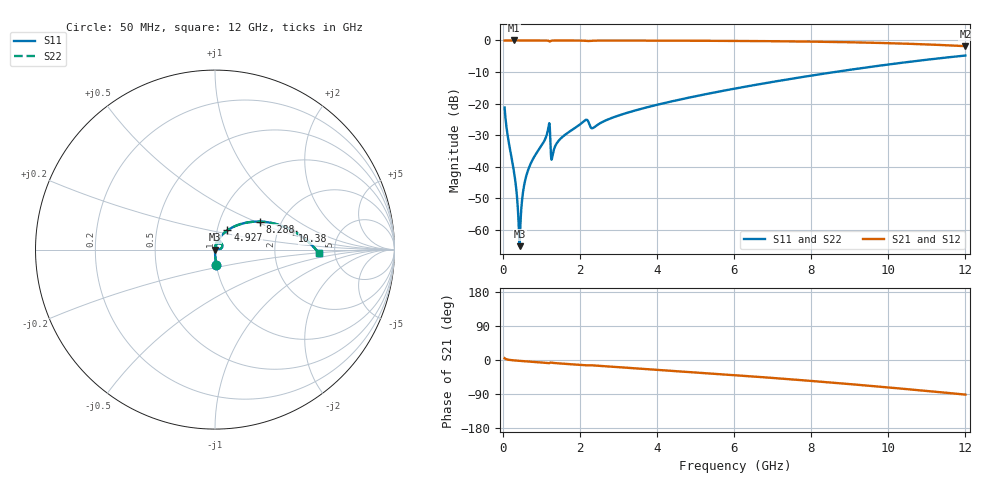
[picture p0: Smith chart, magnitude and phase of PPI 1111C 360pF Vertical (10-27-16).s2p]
# GHz S MA R 50
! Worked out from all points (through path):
!   1601 points, 50 MHz to 12 GHz, reference 50 ohm
!   highest |S21| = 0.00 dB at 289 MHz (marker M1); lowest = -1.8 dB at 12 GHz (marker M2)
!   group delay of S21, straight-line fit = 21 ps
!   lowest |S11| = -65.1 dB at 438.4 MHz (marker M3), VSWR 1.00, Z = 50.1 + j0.00672 ohm
!   |S11| at or under -10 dB: start of sweep to 8.61 GHz
!   |S22| runs from -65.1 to -4.8 dB; largest |S21 - S12| = 0
!   S11 on the Smith chart (normalised r, x): 50 MHz: 1.00, -0.17; 4.927 GHz: 1.12, +0.24; 8.288 GHz: 1.56, +0.53; 10.38 GHz: 2.41, +0.63; 12 GHz: 3.72, -0.19
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0.05  0.08683 -85.1  0.996 4.7  0.996 4.7  0.08683 -85.1
0.289  0.008632 -87.9  0.9995 -1.0  0.9995 -1.0  0.008632 -87.9
0.3412812  0.005086 -85.9  0.9995 -1.5  0.9995 -1.5  0.005086 -85.9
0.3935625  0.00218 -78.0  0.9995 -1.9  0.9995 -1.9  0.00218 -78.0
0.438375  0.0005533 7.0  0.9994 -2.3  0.9994 -2.3  0.0005533 7.0
0.4757188  0.001856 69.7  0.9994 -2.5  0.9994 -2.5  0.001856 69.7
0.557875  0.005153 80.1  0.9993 -3.2  0.9993 -3.2  0.005153 80.1
0.6400313  0.00819 81.7  0.9993 -3.7  0.9993 -3.7  0.00819 81.7
1.162844  0.03572 72.8  0.9936 -8.0  0.9936 -8.0  0.03572 72.8
1.30475  0.01642 68.9  0.996 -7.6  0.996 -7.6  0.01642 68.9
1.498938  0.02778 77.9  0.9981 -9.3  0.9981 -9.3  0.02778 77.9
2.044156  0.04895 72.1  0.9947 -13.2  0.9947 -13.2  0.04895 72.1
2.171125  0.05564 61.2  0.9844 -14.2  0.9844 -14.2  0.05564 61.2
2.350375  0.04133 64.2  0.9908 -14.3  0.9908 -14.3  0.04133 64.2
4.038312  0.09685 63.0  0.9934 -26.0  0.9934 -26.0  0.09685 63.0
4.927094  0.128 57.1  0.9897 -32.1  0.9897 -32.1  0.128 57.1
6.025  0.1731 49.3  0.9825 -40.0  0.9825 -40.0  0.1731 49.3
8.019156  0.2786 34.1  0.9574 -55.4  0.9574 -55.4  0.2786 34.1
8.288031  0.2953 31.9  0.9522 -57.6  0.9522 -57.6  0.2953 31.9
10.01331  0.4169 17.0  0.9051 -72.6  0.9051 -72.6  0.4169 17.0
10.37928  0.4453 13.7  0.8914 -75.9  0.8914 -75.9  0.4453 13.7
12  0.5769 -1.7  0.8121 -91.3  0.8121 -91.3  0.5769 -1.7
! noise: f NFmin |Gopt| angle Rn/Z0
0.05  0.0003432  0.8556  0.3174  0.0005076
1.372  0.005086  0.7488  6.97  0.004061
2.701  0.007612  0.6845  13.53  0.004616
4.031  0.00816  0.5914  19.59  0.00356
5.36  0.009987  0.5707  25.49  0.004018
6.682  0.01195  0.5656  31.09  0.004629
8.012  0.01407  0.5702  36.46  0.005382
9.341  0.0164  0.5824  41.59  0.006317
10.67  0.01903  0.6011  46.53  0.007508
12  0.02206  0.6252  51.31  0.00906
